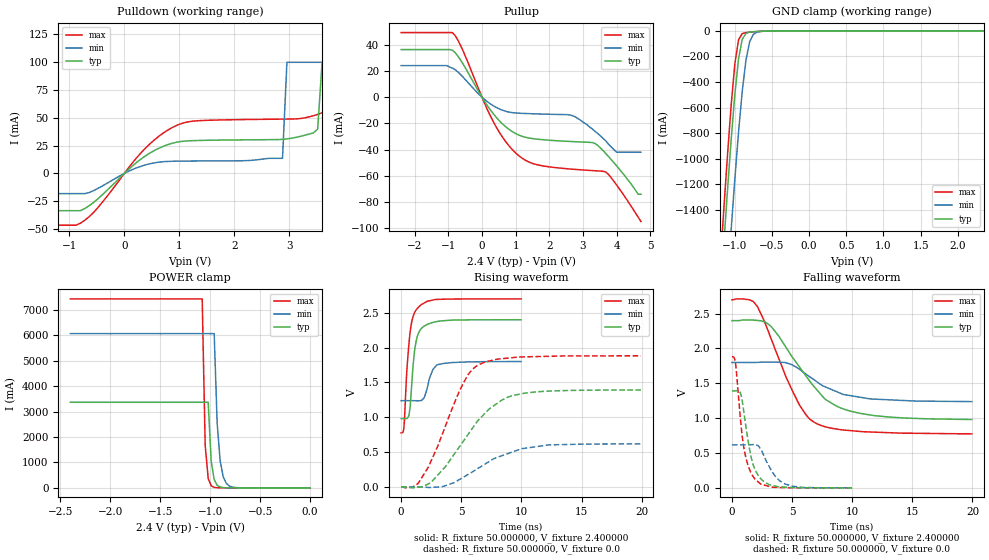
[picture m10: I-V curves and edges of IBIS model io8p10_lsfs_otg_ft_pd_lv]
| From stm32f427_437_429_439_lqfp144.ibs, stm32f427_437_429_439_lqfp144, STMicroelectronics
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|   Model io8p10_lsfs_otg_ft_pd_lv
[Model]  io8p10_lsfs_otg_ft_pd_lv
Model_type I/O
Polarity   Non-Inverting
Enable   Active-Low
Vinl =   0.720000V
Vinh =   1.680000V
Vmeas =  1.200000V
Cref =   40.000000pF
Rref =   100.000000M
Vref =   0.0V
C_comp   7.971100pF   7.737700pF   8.264100pF
[Temperature Range]   25.000000   0.125000k   -40.000000
[Pullup Reference]   2.400000V   1.800000V   2.700000V
[Pulldown Reference]   0.0V   0.0V   0.0V
[POWER Clamp Reference]   2.400000V   1.800000V   2.700000V
[GND Clamp Reference]   0.0V   0.0V   0.0V
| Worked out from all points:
|   slope of the pulldown table from 0 to 0.36 V, typ, clamps not added: 24.1 ohm
|   slope of the pullup table from 0 to 0.36 V, typ, clamps not added: 26.8 ohm
|   GND clamp passes 1 mA (typ) near -0.52 V on its own axis
|   POWER clamp passes 1 mA (typ) near -0.81 V on its own axis
|   rising waveform, R_fixture 50.000000, V_fixture 2.400000: 20-80 % time 481ps typ, 597ps min, 492ps max; typ from 0.981 V to 2.4 V
|   rising waveform, R_fixture 50.000000, V_fixture 0.0: 20-80 % time 3.67ns typ, 4.11ns min, 2.72ns max; typ from 0 V to 1.39 V
|   falling waveform, R_fixture 50.000000, V_fixture 2.400000: 20-80 % time 3.7ns typ, 3.39ns min, 2.85ns max; typ from 2.4 V to 0.981 V
|   falling waveform, R_fixture 50.000000, V_fixture 0.0: 20-80 % time 913ps typ, 1.27ns min, 796ps max; typ from 1.39 V to 0 V
[Pulldown]
|Voltage   I(typ)   I(min)   I(max)
-2.4V     -33.44mA   -18.12mA   -46.52mA
-800mV    -33.44mA   -18.12mA   -44.78mA
1.04V     28.81mA    11.14mA    44.91mA
2.88V     30.7mA     13.64mA    48.89mA
2.96V     31.11mA    100mA      48.94mA
3.52V     40mA       100mA      53.15mA
3.6V      100mA      100mA      54.65mA
3.92V     100mA      100mA      60mA
4V        100mA      100mA      100mA
4.4V      100mA      100mA      100mA
4.48V     100mA      100mA      1A
4.8V      100mA      100mA      1A
[Pullup]
|Voltage   I(typ)   I(min)   I(max)
-2.4V     36.2mA     24mA       49.16mA
-880mV    35.81mA    22.16mA    49.16mA
-640mV    28.47mA    17.31mA    39.62mA
320mV     -12.14mA   -6.322mA   -17.91mA
960mV     -27.18mA   -12mA      -41.54mA
1.52V     -31.65mA   -12.71mA   -50.68mA
2.64V     -33.82mA   -13.73mA   -54.81mA
3.36V     -35.34mA   -26.1mA    -56.1mA
3.68V     -43.1mA    -33.4mA    -57.12mA
4V        -52.4mA    -42mA      -67mA
4.64V     -74mA      -42mA      -91.5mA
4.72V     -74mA      -42mA      -94.8mA
[GND_clamp]
|Voltage   I(typ)   I(min)   I(max)
-2.4V     -9.765A    -9.942A    -9.572A
-1.2V     -2.124A    -2.851A    -1.855A
-1.15V    -1.682A    -2.408A    -1.408A
-1.1V     -1.256A    -1.975A    -979.8mA
-1.05V    -854.9mA   -1.557A    -584.5mA
-1V       -496.5mA   -1.158A    -257.5mA
-950mV    -217.7mA   -789.7mA   -69.53mA
-900mV    -65.58mA   -469.8mA   -21.52mA
-850mV    -19.65mA   -226.4mA   -13.58mA
-800mV    -9.766mA   -84.22mA   -10.49mA
-700mV    -4.935mA   -9.894mA   -5.821mA
2.35V     58.09uA    37.92uA    67.25uA
[POWER_clamp]
|Voltage   I(typ)   I(min)   I(max)
-2.4V     3.365A     6.064A     7.43A
-1.08V    3.365A     6.064A     7.43A
-1.05V    3.365A     6.064A     1.669A
-1.02V    3.365A     6.064A     375mA
-990mV    1.047A     6.064A     84.24mA
-960mV    325.6mA    6.064A     18.93mA
-930mV    101.3mA    2.529A     4.252mA
-900mV    31.51mA    1.055A     955.2uA
-870mV    9.804mA    440.1mA    214.6uA
-840mV    3.05mA     183.6mA    74uA
-720mV    28.58uA    5.557mA    74uA
0V        0A         0A         0A
[Ramp]
| variable   typ   min   max
dV/dt_r  0.83466/3.66668n   0.37030/4.10403n   1.12872/2.71995n
dV/dt_f  0.84756/3.69409n   0.33672/3.41934n   1.15378/2.85235n
R_load = 50.000000
[Rising Waveform]
R_fixture= 50.000000
V_fixture= 2.400000
V_fixture_min= 1.800000
V_fixture_max= 2.700000
|time   V(typ)   V(min)   V(max)
0s        980.6mV    1.238V     774.7mV
220.2ps   980.3mV    1.238V     836.5mV
440.4ps   981.7mV    1.238V     1.574V
640.6ps   1.021V     1.238V     2.038V
820.8ps   1.322V     1.238V     2.313V
1.101ns   1.935V     1.237V     2.495V
1.421ns   2.198V     1.236V     2.576V
1.922ns   2.308V     1.281V     2.64V
2.963ns   2.372V     1.748V     2.691V
9.97ns    2.399V     1.799V     2.699V
[Rising Waveform]
R_fixture= 50.000000
V_fixture= 0.0
V_fixture_min= 0.0
V_fixture_max= 0.0
|time   V(typ)   V(min)   V(max)
0s        15.03uV    7.253uV    -90.55uV
1.441ns   -5.115mV   71.56uV    56.85mV
2.482ns   63.79mV    -7.425mV   369.3mV
3.483ns   252.8mV    6.391mV    784.4mV
5.165ns   654.2mV    138.1mV    1.487V
5.766ns   801.9mV    199.3mV    1.655V
6.527ns   976.4mV    280mV      1.76V
8.368ns   1.246V     447mV      1.84V
10.21ns   1.343V     553.1mV    1.866V
19.94ns   1.391V     617.3mV    1.881V
[Falling Waveform]
R_fixture= 50.000000
V_fixture= 2.400000
V_fixture_min= 1.800000
V_fixture_max= 2.700000
|time   V(typ)   V(min)   V(max)
0s        2.399V     1.799V     2.699V
1.441ns   2.408V     1.799V     2.699V
2.122ns   2.402V     1.8V       2.6V
3.243ns   2.318V     1.803V     2.145V
5.125ns   1.851V     1.752V     1.356V
6.126ns   1.612V     1.636V     1.055V
6.967ns   1.425V     1.533V     928.7mV
8.769ns   1.167V     1.375V     841.9mV
10.77ns   1.066V     1.297V     807.1mV
19.94ns   980.6mV    1.238V     774.7mV
[Falling Waveform]
R_fixture= 50.000000
V_fixture= 0.0
V_fixture_min= 0.0
V_fixture_max= 0.0
|time   V(typ)   V(min)   V(max)
0s        1.391V     617.3mV    1.881V
300.3ps   1.393V     617.3mV    1.777V
760.8ps   1.328V     617.2mV    887.3mV
1.041ns   1.022V     616.9mV    526.4mV
1.562ns   462.4mV    618.6mV    223.3mV
1.922ns   262.4mV    620.3mV    122.3mV
2.683ns   85.94mV    450.2mV    39.62mV
3.624ns   24.66mV    160.4mV    7.244mV
4.404ns   9.149mV    55.87mV    3.21mV
9.97ns    15.03uV    7.253uV    -90.55uV
